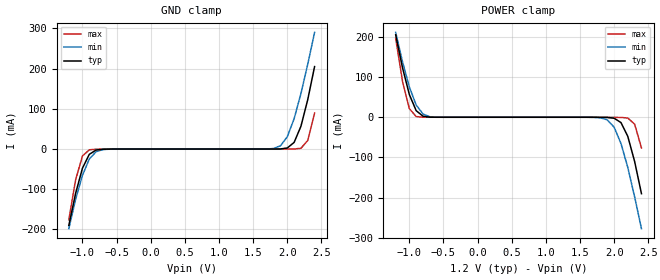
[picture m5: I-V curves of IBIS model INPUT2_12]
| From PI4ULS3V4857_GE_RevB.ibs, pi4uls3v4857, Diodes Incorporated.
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[Model] INPUT2_12
Model_type Input
Vinl = 0.24V
Vinh = 0.96V
| variable   typ   min   max
C_comp   0.832pF   0.829pF   0.836pF
[Voltage Range]   1.2V   1.1V   1.3V
[GND Clamp Reference]   0.000V   0.000V   0.000V
[POWER Clamp Reference]   1.2V   1.1V   1.3V
[temperature range]   40   85   -40
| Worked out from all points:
|   GND clamp passes 1 mA (typ) near -0.73 V on its own axis
|   POWER clamp passes 1 mA (typ) near -0.73 V on its own axis
[GND Clamp]
| Voltage   I(typ)   I(min)   I(max)
-1.2V     -190mA     -198mA     -176mA
-1.1V     -110mA     -125mA     -76.3mA
-1V       -47.6mA    -65.3mA    -17.2mA
-900mV    -13.2mA    -24.9mA    -2.01mA
-800mV    -2.5mA     -6.63mA    -466uA
1.7V      5.04uA     112uA      4.75uA
1.9V      191uA      8.06mA     5.31uA
2V        2.58mA     30.5mA     5.89uA
2.1V      16.4mA     75.3mA     41.5uA
2.2V      56.5mA     138mA      1.78mA
2.3V      123mA      211mA      21.4mA
2.4V      205mA      290mA      89.4mA
[POWER Clamp]   |Note: Vtable = Vcc - Voutput
| Voltage   I(typ)   I(min)   I(max)
-1.2V     205mA      211mA      196mA
-1.1V     123mA      138mA      89.4mA
-1V       56.5mA     75.3mA     21.4mA
-900mV    16.4mA     30.5mA     1.78mA
-800mV    2.58mA     8.06mA     41.5uA
-600mV    11.6uA     112uA      5.31uA
1.9V      -488uA     -6.63mA    -113uA
2V        -2.5mA     -24.9mA    -265uA
2.1V      -13.2mA    -65.3mA    -466uA
2.2V      -47.6mA    -125mA     -2.01mA
2.3V      -110mA     -198mA     -17.2mA
2.4V      -190mA     -277mA     -76.3mA
